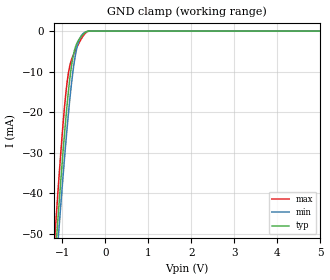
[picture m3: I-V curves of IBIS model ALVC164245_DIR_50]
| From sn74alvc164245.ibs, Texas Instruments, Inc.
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[Model]   ALVC164245_DIR_50
Model_type  Input
Vinl = 0.8
Vinh = 2
| variable   typ   min   max
C_comp   6.5pF   NA   NA
[Temperature Range]   40   100   -40
| Ambient temperature   25   85   -40
[Voltage range]   5   4.5   5.5
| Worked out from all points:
|   GND clamp passes 1 mA (typ) near -0.53 V on its own axis
[GND Clamp]
| ALVC164245_DIR_50
|   Voltage   I(typ)   I(min)   I(max)
-5V       -702.4mA   -687.9mA   -721.5mA
-1.18V    -57.67mA   -63.23mA   -51.41mA
-1.135V   -50.94mA   -56.66mA   -44.41mA
-1.095V   -45.07mA   -50.93mA   -38.33mA
-1.075V   -42.19mA   -48.1mA    -35.37mA
-920mV    -21.52mA   -27.44mA   -15.38mA
-860mV    -14.84mA   -20.33mA   -10.36mA
-790mV    -8.686mA   -13.06mA   -7.132mA
-720mV    -4.776mA   -7.342mA   -5.312mA
-645mV    -2.623mA   -3.355mA   -3.612mA
-460mV    -307.5uA   -191uA     -475.8uA
5V        919.4pA    48.35nA    20.01pA
